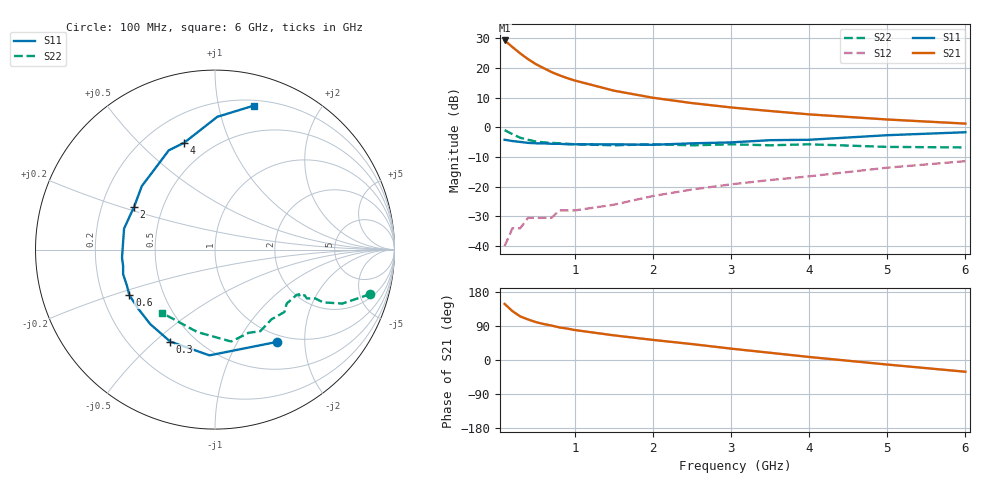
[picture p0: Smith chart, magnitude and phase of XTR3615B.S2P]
! HXTR-3615 Common Emitter
! Vce=15V  Ic=18mA
# ghz s ma r 50
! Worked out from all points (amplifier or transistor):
!   18 points, 100 MHz to 6 GHz, reference 50 ohm
!   highest |S21| = 29.3 dB at 100 MHz (marker M1)
!   |S21| within 3 dB of that: start of sweep to 236.6 MHz
!   unconditionally stable (mu >= 1): 1.128 GHz to 2.536 GHz
!   at 400 MHz: K = 0.46, MSG = 26.7 dB, |S12| = -30.5 dB
!   at 1 GHz: K = 0.95, MSG = 21.9 dB, |S12| = -28.0 dB
!   at 6 GHz: K = 0.35, MSG = 6.3 dB, |S12| = -11.4 dB
!   S11 on the Smith chart (normalised r, x): 100 MHz: 0.89, -1.49; 300 MHz: 0.37, -0.56; 600 MHz: 0.32, -0.23; 2 GHz: 0.34, +0.22; 4 GHz: 0.36, +0.69; 6 GHz: 0.25, +1.27
0.1  0.62 -56.0  29.17 148.0  0.01 69.0  0.9 -16.0
0.2  0.59 -93.0  22.6 129.0  0.02 66.0  0.77 -23.0
0.3  0.57 -116.0  17.66 115.0  0.02 50.0  0.67 -26.0
0.4  0.55 -131.0  14.14 107.0  0.03 55.0  0.62 -26.0
0.5  0.54 -143.0  11.65 100.0  0.03 47.0  0.58 -28.0
0.6  0.54 -152.0  9.96 95.0  0.03 48.0  0.56 -27.0
0.7  0.53 -158.0  8.57 91.0  0.03 51.0  0.55 -28.0
0.8  0.53 -165.0  7.57 86.0  0.04 52.0  0.54 -29.0
0.9  0.52 -170.0  6.78 83.0  0.04 57.0  0.53 -28.0
1  0.52 -175.0  6.16 79.0  0.04 57.0  0.52 -29.0
1.5  0.52 167.0  4.16 65.0  0.05 59.0  0.5 -37.0
2  0.51 152.0  3.16 53.0  0.07 63.0  0.52 -42.0
2.5  0.54 139.0  2.57 42.0  0.09 64.0  0.5 -51.0
3  0.56 127.0  2.17 30.0  0.11 62.0  0.52 -61.0
3.5  0.61 115.0  1.89 19.0  0.13 59.0  0.5 -68.0
4  0.62 106.0  1.66 8.0  0.15 55.0  0.52 -80.0
5  0.74 89.0  1.36 -12.0  0.21 45.0  0.47 -102.0
6  0.83 75.0  1.16 -31.0  0.27 34.0  0.46 -130.0
